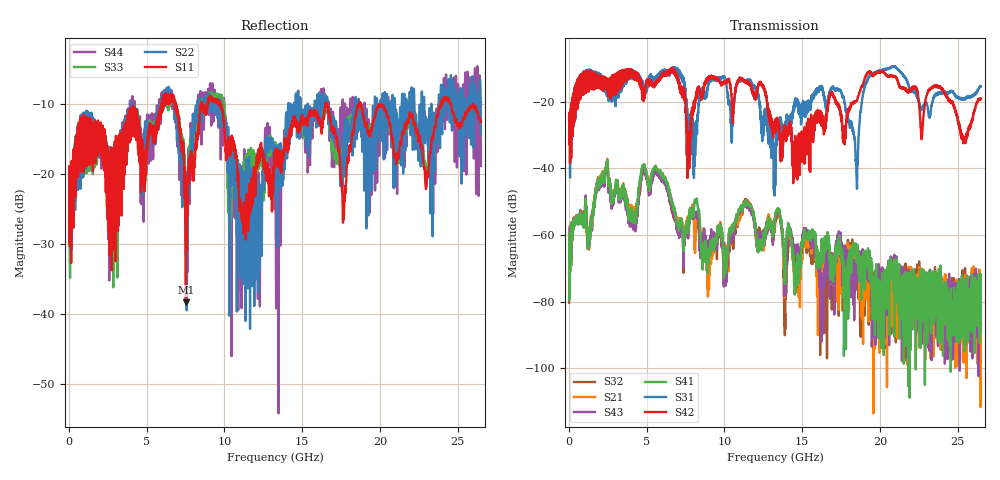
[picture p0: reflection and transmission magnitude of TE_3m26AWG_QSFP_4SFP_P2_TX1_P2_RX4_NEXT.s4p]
!Agilent Technologies,N5222A,MY51421691,A.10.00.00
!Agilent N5222A: A.10.00.00
!Date: Friday, January 30, 2015 12:36:05
!Correction: S11(Full 4 Port(1,2,3,4))
!S12(Full 4 Port(1,2,3,4))
!S13(Full 4 Port(1,2,3,4))
!S14(Full 4 Port(1,2,3,4))
!S21(Full 4 Port(1,2,3,4))
!S22(Full 4 Port(1,2,3,4))
!S23(Full 4 Port(1,2,3,4))
!S24(Full 4 Port(1,2,3,4))
!S31(Full 4 Port(1,2,3,4))
!S32(Full 4 Port(1,2,3,4))
!S33(Full 4 Port(1,2,3,4))
!S34(Full 4 Port(1,2,3,4))
!S41(Full 4 Port(1,2,3,4))
!S42(Full 4 Port(1,2,3,4))
!S43(Full 4 Port(1,2,3,4))
!S44(Full 4 Port(1,2,3,4))
!S4P File: Measurements: <S11,S12,S13,S14>,
!<S21,S22,S23,S24>,
!<S31,S32,S33,S34>,
!<S41,S42,S43,S44>:
# Hz S  dB  R 50.0
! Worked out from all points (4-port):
!   2650 points, 10 MHz to 26.5 GHz, reference 50 ohm
!   strongest paths, dB at 10 MHz, 6.63 GHz, 13.26 GHz, 19.88 GHz, 26.5 GHz:
!     S42: -24.9, -10.9, -25.3, -11.1, -19.0
!     S31: -24.9, -10.3, -36.2, -10.7, -15.2
!     S41: -68.6, -50.4, -54.6, -74.6, -71.8
!     S43: -71.9, -52.5, -55.0, -76.9, -81.8
!     S21: -71.5, -50.9, -55.7, -87.2, -88.0
!     S32: -80.3, -53.3, -56.6, -77.6, -81.1
!   lowest |S11| = -38.3 dB at 7.52 GHz (marker M1), VSWR 1.02, Z = 51.2 + j0.274 ohm
!   |S11| at or under -10 dB: start of sweep to 5.956 GHz; 9.72 GHz to 16.5 GHz (6.776 GHz wide, 51.7 % of centre); 18.73 GHz to 23.92 GHz (5.186 GHz wide, 24.3 % of centre)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
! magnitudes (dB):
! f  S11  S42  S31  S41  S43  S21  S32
! 10 MHz  -18.9  -24.9  -24.9  -68.6  -71.9  -71.5  -80.3
! 2.38 GHz  -16.3  -12.9  -13.1  -40.3  -41.4  -40.2  -41.3
! 7.52 GHz  -38.3  -21.7  -19.8  -57.3  -58.6  -57.4  -57.8
! 17.33 GHz  -16.7  -20.9  -16.4  -61.1  -60.5  -74.1  -76.6
! 18.49 GHz  -11.1  -19.9  -41.7  -64.1  -68.9  -63.5  -75.4
! 19.59 GHz  -12.3  -12.3  -11.4  -74.9  -82.5  -75.6  -77.7
! 26.5 GHz  -12.6  -19.0  -15.2  -71.8  -81.8  -88.0  -81.1
